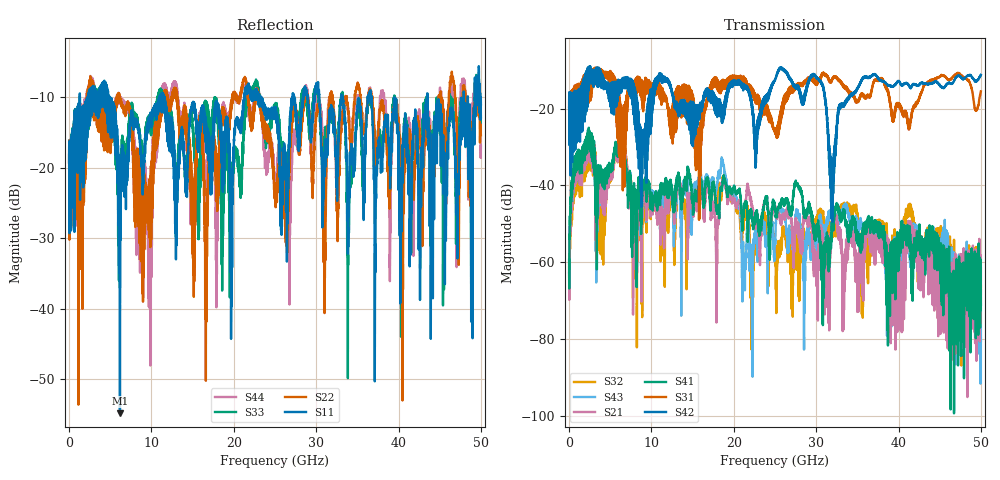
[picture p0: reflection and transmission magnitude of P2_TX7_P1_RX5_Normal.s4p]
!Keysight Technologies,N5225B,MY57041031,A.13.20.10
!Date: Friday, May 31, 2019 11:21:58
!Correction: S11(Full 4 Port(1,2,3,4))
!S12(Full 4 Port(1,2,3,4))
!S13(Full 4 Port(1,2,3,4))
!S14(Full 4 Port(1,2,3,4))
!S21(Full 4 Port(1,2,3,4))
!S22(Full 4 Port(1,2,3,4))
!S23(Full 4 Port(1,2,3,4))
!S24(Full 4 Port(1,2,3,4))
!S31(Full 4 Port(1,2,3,4))
!S32(Full 4 Port(1,2,3,4))
!S33(Full 4 Port(1,2,3,4))
!S34(Full 4 Port(1,2,3,4))
!S41(Full 4 Port(1,2,3,4))
!S42(Full 4 Port(1,2,3,4))
!S43(Full 4 Port(1,2,3,4))
!S44(Full 4 Port(1,2,3,4))
!S4P File: Measurements: <S11,S12,S13,S14>,
!<S21,S22,S23,S24>,
!<S31,S32,S33,S34>,
!<S41,S42,S43,S44>:
# Hz S  dB  R 50.0
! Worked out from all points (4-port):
!   5000 points, 10 MHz to 50 GHz, reference 50 ohm
!   strongest paths, dB at 10 MHz, 12.51 GHz, 25.01 GHz, 37.51 GHz, 50 GHz:
!     S42: -19.6, -15.5, -12.6, -12.0, -11.2
!     S31: -19.7, -21.1, -25.8, -12.7, -15.5
!     S41: -59.4, -40.8, -45.8, -51.0, -71.0
!     S21: -62.6, -42.1, -45.2, -52.9, -61.6
!     S43: -63.1, -41.1, -54.1, -53.0, -80.6
!     S32: -61.3, -43.0, -57.1, -51.9, -66.2
!   lowest |S11| = -54.8 dB at 6.18 GHz (marker M1), VSWR 1.00, Z = 50.1 - j0.161 ohm
!   |S11| at or under -10 dB: 4.96 GHz to 11.03 GHz (6.067 GHz wide, 75.9 % of centre); 11.57 GHz to 21.26 GHz (9.683 GHz wide, 59 % of centre); 43.5 GHz to 47.91 GHz (4.402 GHz wide, 9.63 % of centre)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
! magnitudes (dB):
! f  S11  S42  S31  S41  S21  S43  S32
! 10 MHz  -19.3  -19.6  -19.7  -59.4  -62.6  -63.1  -61.3
! 820 MHz  -15.8  -18.5  -16.5  -32.8  -35.2  -35.0  -37.7
! 6.18 GHz  -54.8  -13.4  -18.2  -29.1  -29.7  -29.4  -30.1
! 29.78 GHz  -9.9  -11.1  -12.5  -51.4  -60.3  -57.6  -50.0
! 31.9 GHz  -12.0  -38.3  -12.7  -49.5  -50.8  -47.9  -51.5
! 35.81 GHz  -21.1  -11.7  -16.7  -52.1  -57.0  -51.4  -57.8
! 50 GHz  -11.0  -11.2  -15.5  -71.0  -61.6  -80.6  -66.2
